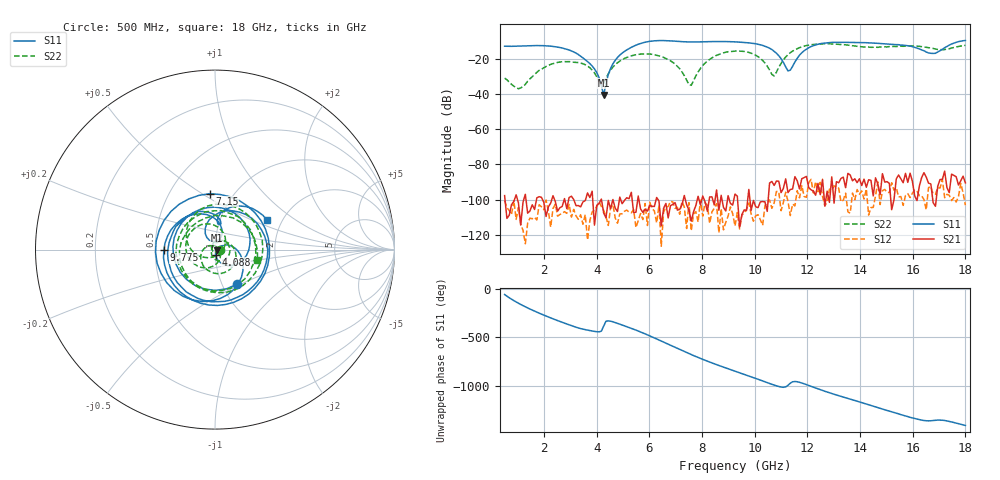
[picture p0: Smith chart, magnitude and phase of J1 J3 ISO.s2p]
!Agilent Technologies,N5230A,MY45001360,A.07.50.67
!Agilent N5230A: A.07.50.67
!Date: Tuesday, April 16, 2024 16:25:21
!Correction: S11(Full 2 Port(1,2))
!S21(Full 2 Port(1,2))
!S12(Full 2 Port(1,2))
!S22(Full 2 Port(1,2))
!S2P File: Measurements: S11, S21, S12, S22:
# Hz S  dB  R 50
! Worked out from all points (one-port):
!   201 points, 500 MHz to 18 GHz, reference 50 ohm
!   lowest |S11| = -40.5 dB at 4.263 GHz (marker M1), VSWR 1.02, Z = 50.9 - j0.367 ohm
!   |S11| at or under -10 dB: start of sweep to 6.024 GHz; 7.025 GHz to 17.8 GHz (10.77 GHz wide, 86.8 % of centre)
!   S11 on the Smith chart (normalised r, x): 500 MHz: 1.18, -0.48; 4.088 GHz: 1.01, -0.06; 7.15 GHz: 0.78, +0.54; 9.775 GHz: 0.56, -0.01; 18 GHz: 1.67, +0.62
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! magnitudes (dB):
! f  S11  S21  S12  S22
! 500 MHz  -12.8  -97.8  -100.6  -31.0
! 1.025 GHz  -12.7  -101.9  -104.5  -37.0
! 2.25 GHz  -12.8  -102.0  -115.7  -23.1
! 3.475 GHz  -19.5  -101.4  -114.1  -22.8
! 4.088 GHz  -30.7  -102.2  -101.1  -32.6
! 4.263 GHz  -40.5  -107.7  -106.1  -33.8
! 4.525 GHz  -25.4  -105.2  -104.6  -26.4
! 4.875 GHz  -17.9  -98.6  -108.2  -21.3
! 6.362 GHz  -9.6  -100.8  -103.3  -18.3
! 7.15 GHz  -10.1  -105.6  -108.4  -25.6
! 7.588 GHz  -10.4  -112.3  -117.7  -35.0
! 8.2 GHz  -10.2  -106.7  -103.1  -21.3
! 9.25 GHz  -10.3  -96.9  -115.1  -15.6
! 9.775 GHz  -10.9  -94.3  -102.0  -16.3
! 10.21 GHz  -12.0  -101.3  -111.5  -19.7
! 10.74 GHz  -15.7  -92.0  -101.8  -29.7
! 11.26 GHz  -26.9  -96.0  -101.1  -17.6
! 11.79 GHz  -16.5  -88.1  -92.1  -13.2
! 12.22 GHz  -12.5  -95.2  -96.3  -11.9
! 15.11 GHz  -11.7  -90.9  -96.0  -13.0
! 16.86 GHz  -16.8  -103.8  -97.0  -14.3
! 18 GHz  -9.5  -90.5  -103.3  -12.3
